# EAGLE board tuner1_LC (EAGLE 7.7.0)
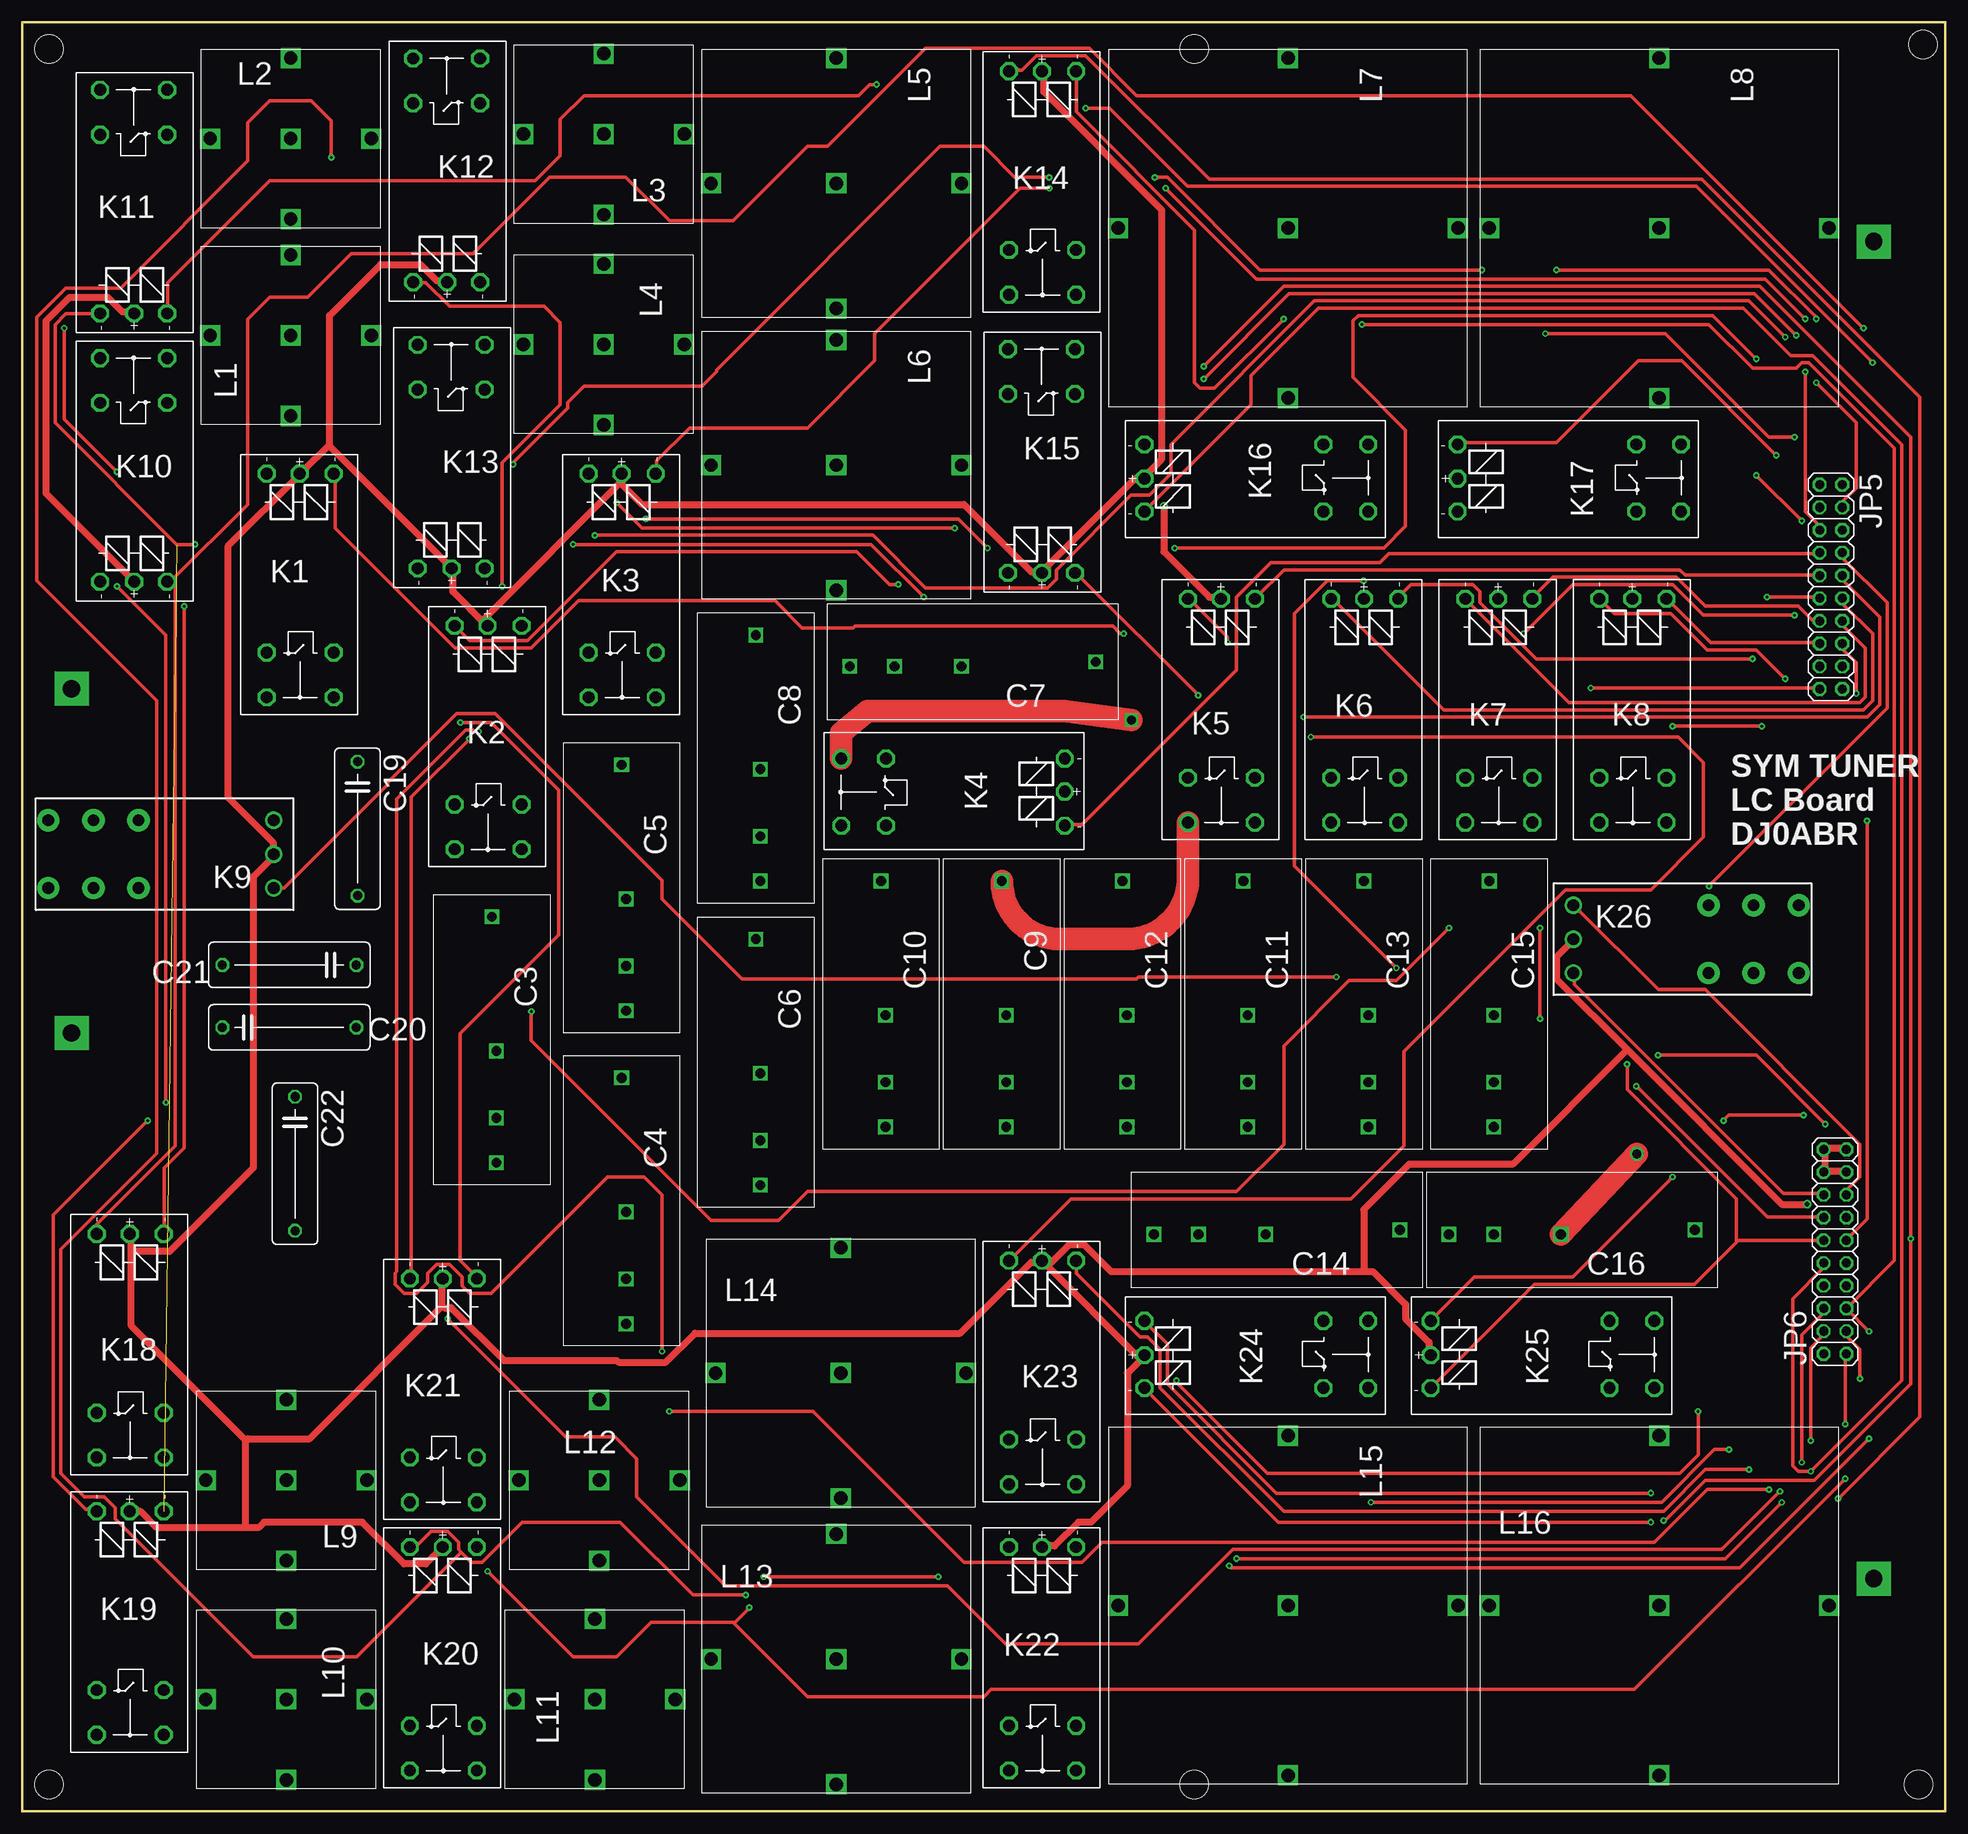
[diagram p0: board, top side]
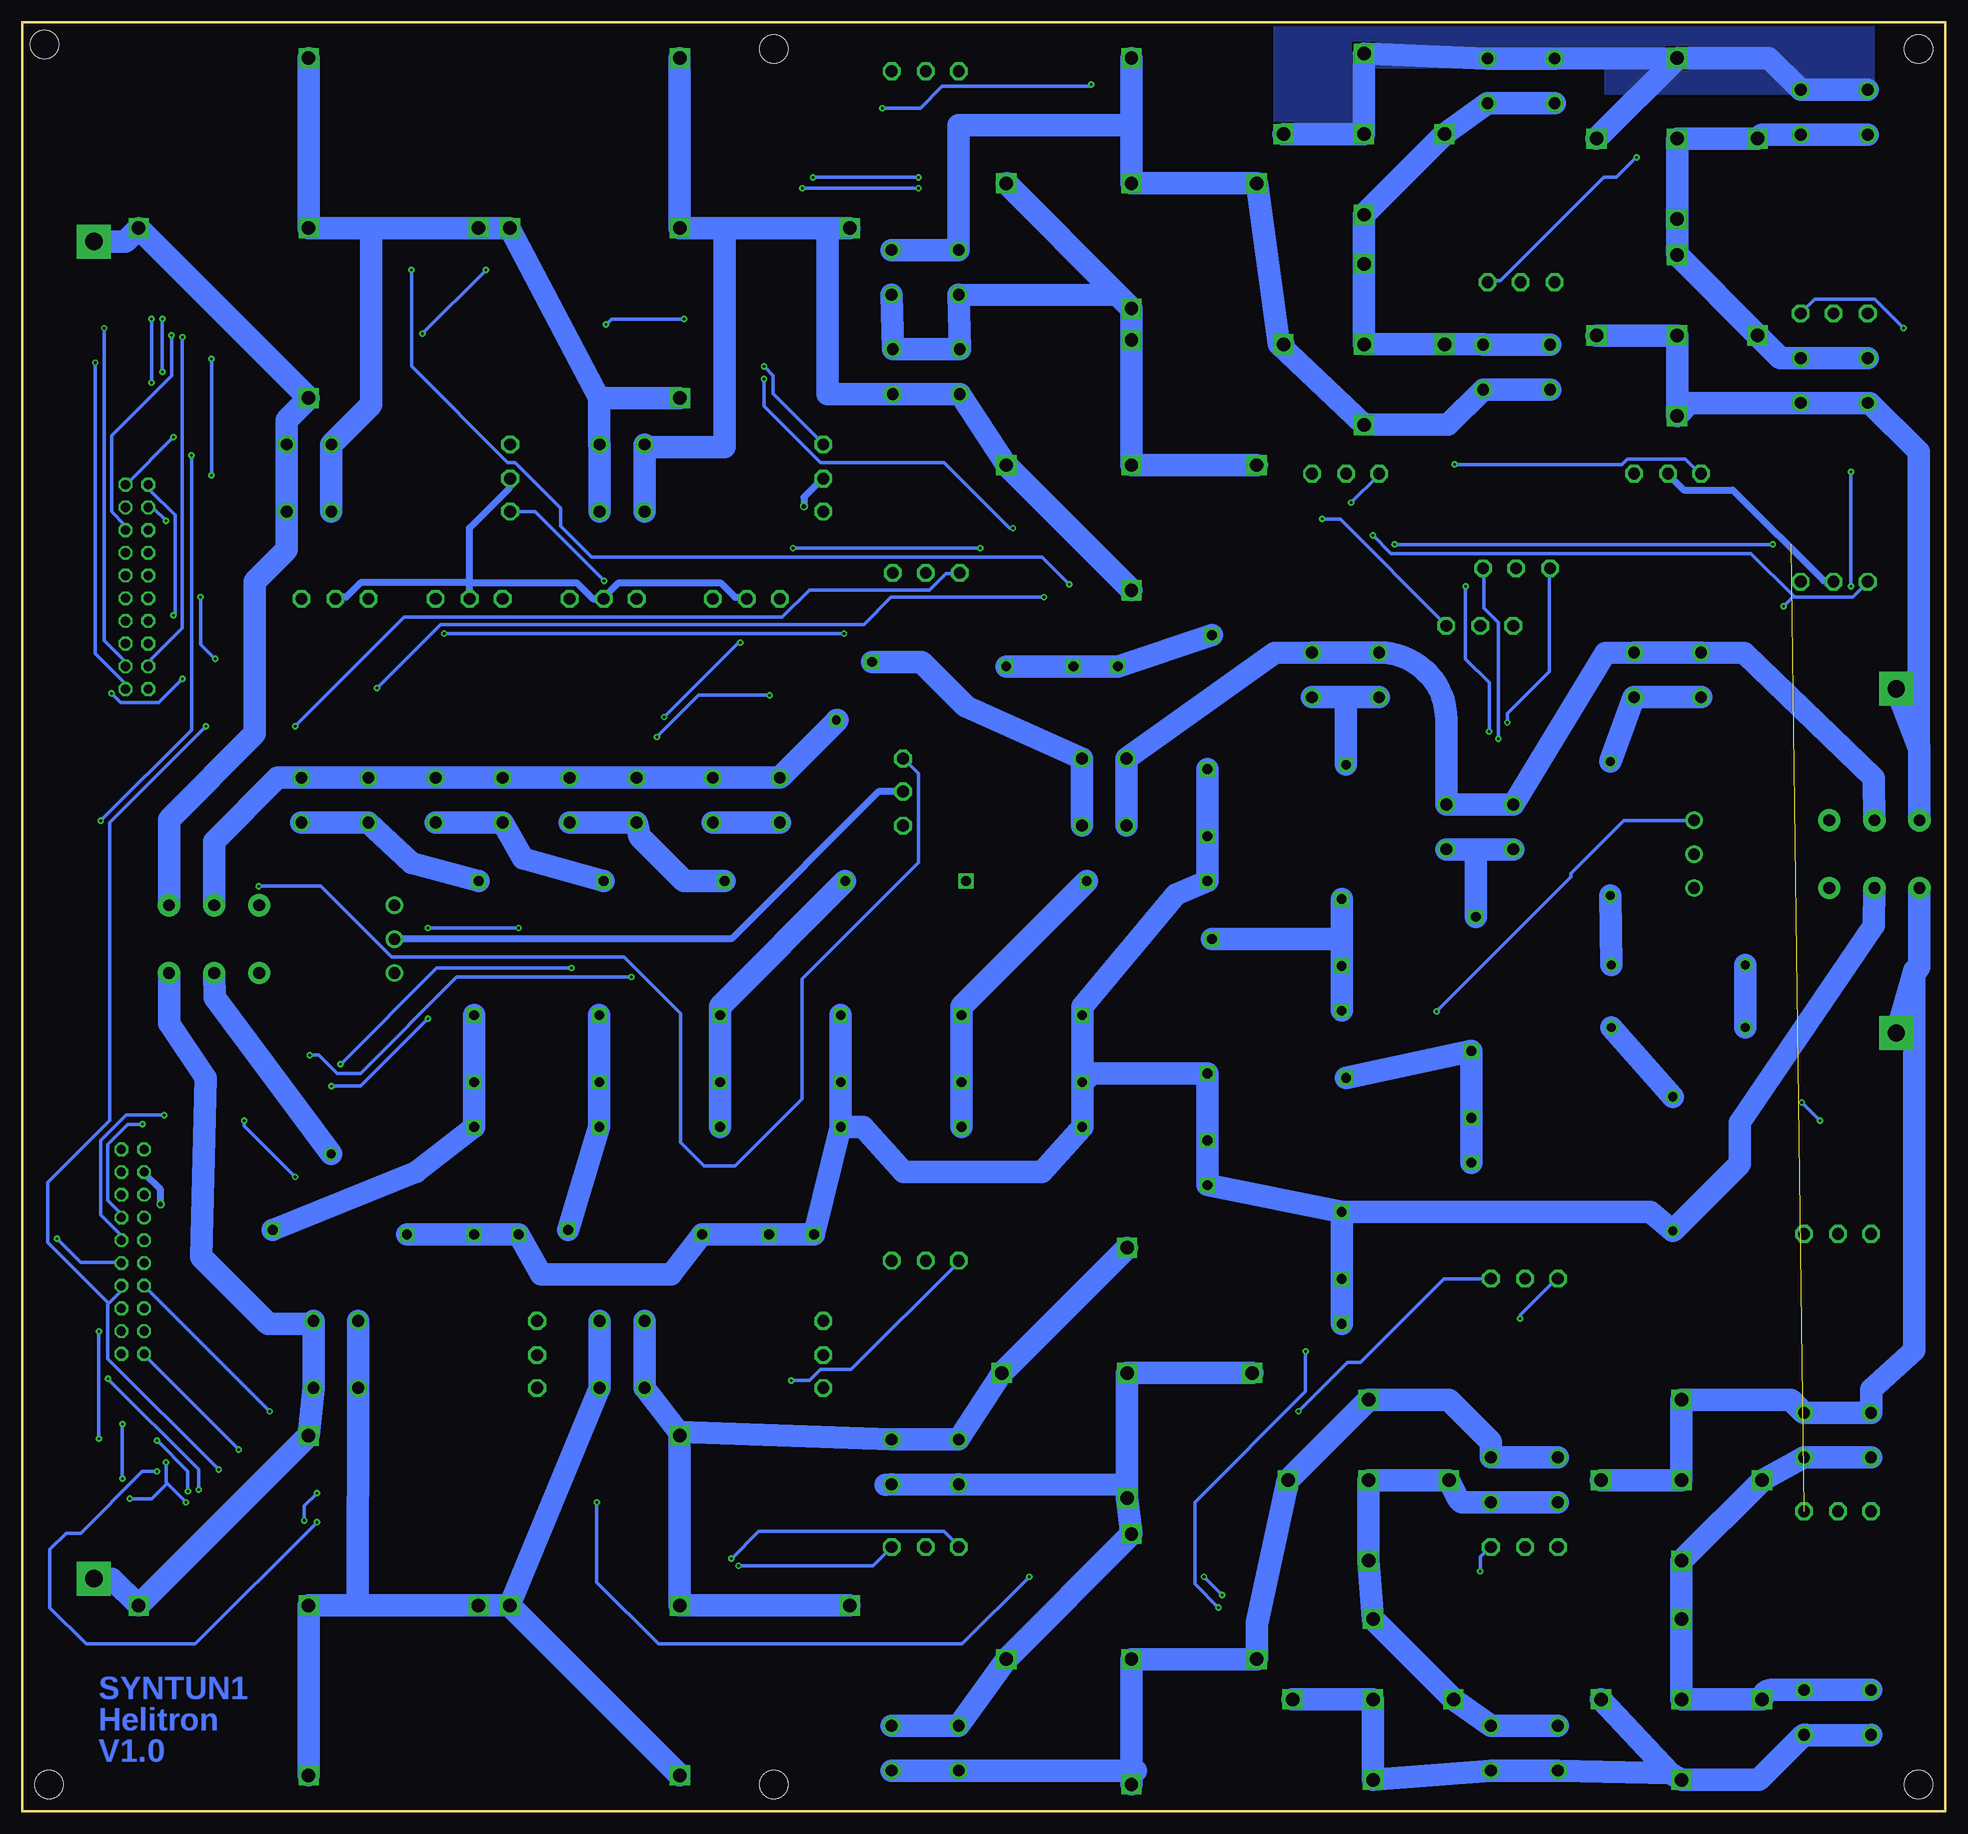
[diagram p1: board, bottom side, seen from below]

Size 215 x 200 mm. Coordinates in mm from the lower left corner, seen from the top.
Outline: 0,0 215,0 215,200 0,200 0,0
Copper layers (1*16): Top 0.035mm / dielectric 1.5mm / Bottom 0.035mm
Design rules "default *": minimum track width 16mil, minimum drill 0.3mm, track to track 16mil, track to pad 16mil, pad to pad 16mil, via to via 16mil, smd to smd 0mil, copper to edge 10mil, drill to drill 8mil, minimum pad ring 10mil, minimum via ring 8mil, stop-mask expansion 4mil, vias tented up to drill 0mil, thermal gap 10mil
Net classes: 1 Supply: width 0.762 mm, drill 0.5 mm; 2 HF: width 2.5 mm, drill 1 mm, clearance 2.5 mm
Holes 3.2 mm at 3,3 3,197 212.5,197.5 212,3 131,3 131,197

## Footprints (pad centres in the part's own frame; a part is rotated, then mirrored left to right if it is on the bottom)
C_FKP_MULTI = drill 1.1 square: 1 0,0; 2A 15,0.5; 2B 22.5,0.5; 2C 27.5,0.5
C150-054X183 = drill 1.016 octagon: 1 -7.493,0; 2 7.493,0
THICKPIN = drill 1.93 pad 3.81 square: 1 0,0
2X10 = drill 1.016 octagon: 1 -11.43,-1.27; 2 -11.43,1.27; 3 -8.89,-1.27; 4 -8.89,1.27; 5 -6.35,-1.27; 6 -6.35,1.27; 7 -3.81,-1.27; 8 -3.81,1.27; 9 -1.27,-1.27; 10 -1.27,1.27; 11 1.27,-1.27; 12 1.27,1.27; 13 3.81,-1.27; 14 3.81,1.27; 15 6.35,-1.27; 16 6.35,1.27; 17 8.89,-1.27; 18 8.89,1.27; 19 11.43,-1.27; 20 11.43,1.27
G2RLK1A = drill 1.321 octagon: 1 -2.54,-3.683; 2 -2.54,3.81; 3 -2.54,0; P 17.45,-3.683; P@ 17.45,3.81; S 22.454,-3.683; S@ 22.454,3.81
RT424 = drill 1.3 pad 2.5: 11 7.56,-3.78; 12 2.52,-3.78; 14 12.6,-3.78; 21 7.56,3.78; 22 2.52,3.78; 24 12.6,3.78 | drill 1.3: A1 -12.6,-3.78; A2 -12.6,3.78; A3 -12.6,0
L_D20 = drill 1.5 square: 1A 1,0; 1B 10,0; 1C 10,-9; 2A 19,0; 2B 10,9
L_D30 = drill 1.5 square: 1A 1,0; 1B 15,0; 1C 15,-14; 2A 29,0; 2B 15,14
L_D40 = drill 1.5 square: 1A 1,0; 1B 20,0; 1C 20,-19; 2A 39,0; 2B 20,19

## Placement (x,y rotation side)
C3  100p  [C_FKP_MULTI]  52.5,100 270 top
C4  100p  [C_FKP_MULTI]  67,82 270 top
C5  150p  [C_FKP_MULTI]  67,117 270 top
C6  220p  [C_FKP_MULTI]  82,97.5 270 top
C7  330p  [C_FKP_MULTI]  120,128.5 180 top
C8  330p  [C_FKP_MULTI]  82,131.5 270 top
C9  680p  [C_FKP_MULTI]  109.5,104 270 top
C10  680p  [C_FKP_MULTI]  96,104 270 top
C11  1n  [C_FKP_MULTI]  136.5,104 270 top
C12  1n5  [C_FKP_MULTI]  123,104 270 top
C13  1n5  [C_FKP_MULTI]  150,104 270 top
C14  4n7  [C_FKP_MULTI]  154,65 180 top
C15  3n3  [C_FKP_MULTI]  164,104 270 top
C16  4n7  [C_FKP_MULTI]  187,65 180 top
C19  100p  [C150-054X183]  37.47,109.86 270 top
C20  100p  [C150-054X183]  29.84,94.61 180 top
C21  100p  [C150-054X183]  29.84,87.63 0 top
C22  100p  [C150-054X183]  30.48,72.39 270 top
JP1  [THICKPIN]  5.5,125.5 0 top
JP2  [THICKPIN]  5.5,87 0 top
JP3  [THICKPIN]  207,175.5 0 top
JP4  [THICKPIN]  207,26 0 top
JP5  [2X10]  202.2,136.89 270 top
JP6  [2X10]  202.66,62.56 90 top
K1  G5RLK1AEDC12  [G2RLK1A]  31,147 270 top
K2  G5RLK1AEDC12  [G2RLK1A]  52,130 270 top
K3  G5RLK1AEDC12  [G2RLK1A]  67,147 270 top
K4  G5RLK1AEDC12  [G2RLK1A]  114,114 180 top
K5  G5RLK1AEDC12  [G2RLK1A]  134,133 270 top
K6  G5RLK1AEDC12  [G2RLK1A]  150,133 270 top
K7  G5RLK1AEDC12  [G2RLK1A]  165,133 270 top
K8  G5RLK1AEDC12  [G2RLK1A]  180,133 270 top
K9  RT424F12  [RT424]  15.5,107 180 top
K10  [G2RLK1A]  12.5,140 90 top
K11  [G2RLK1A]  12.5,170 90 top
K12  [G2RLK1A]  47.5,173.5 90 top
K13  [G2RLK1A]  48,141.5 90 top
K14  [G2RLK1A]  114,192 270 top
K15  [G2RLK1A]  114,141 90 top
K16  [G2RLK1A]  128,149 0 top
K17  [G2RLK1A]  163,149 0 top
K18  [G2RLK1A]  12,62 270 top
K19  [G2RLK1A]  12,31 270 top
K20  [G2RLK1A]  47,27 270 top
K21  [G2RLK1A]  47,57 270 top
K22  [G2RLK1A]  114,27 270 top
K23  [G2RLK1A]  114,59 270 top
K24  [G2RLK1A]  128,51 0 top
K25  [G2RLK1A]  160,51 0 top
K26  RT424F12  [RT424]  186,97.5 0 top
L1  187nH  [L_D20]  30,155 90 top
L2  375nH  [L_D20]  20,187 0 top
L3  750nH  [L_D20]  75,187.5 180 top
L4  1,5uH  [L_D20]  65,174 270 top
L5  3uH  [L_D30]  91,197 270 top
L6  6uH  [L_D30]  91,165.5 270 top
L7  12uH  [L_D40]  141.5,197 270 top
L8  24uH  [L_D40]  183,197 270 top
L9  187nH  [L_D20]  39.5,37 180 top
L10  375nH  [L_D20]  29.5,22.5 270 top
L11  750nH  [L_D20]  64,2.5 90 top
L12  1,5uH  [L_D20]  54.5,37 0 top
L13  3uH  [L_D30]  76,17 0 top
L14  6uH  [L_D30]  76.5,49 0 top
L15  12uH  [L_D40]  141.5,43 270 top
L16  24uH  [L_D40]  163,23 0 top

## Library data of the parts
C3-C16 L1-L16 = km_HF
C19-C22 = rcl
JP1-JP4 = km
JP5 JP6 = pinhead
K1-K8 K10-K25 = km; OC_FARNELL: unknown; OC_NEWARK: unknown
K9 K26 = relay; OC_FARNELL: unknown; OC_NEWARK: unknown

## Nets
+12V [Supply]: JP6.17 JP6.18 JP6.19 JP6.20 K1.3 K2.3 K3.3 K4.3 K5.3 K6.3 K7.3 K8.3 K9.A3 K10.3 K11.3 K12.3 K13.3 K14.3 K15.3 K16.3 K17.3 K18.3 K19.3 K20.3 K21.3 K22.3 K23.3 K24.3 K25.3 K26.A3
N$1 [HF]: C19.1 K1.S K1.S@
N$3 [HF]: C3.1 K2.S K2.S@
N$4 [HF]: C3.2A C3.2B C3.2C C4.1
N$5 [HF]: C5.1 K3.S K3.S@
N$6 [HF]: C5.2A C5.2B C5.2C C6.1
N$7 [HF]: C7.1 K4.P K4.P@
N$8 [HF]: C7.2A C7.2B C7.2C C8.1
N$9 [HF]: C9.1 K5.S K5.S@
N$10 [HF]: C9.2A C9.2B C9.2C C10.1
N$11 [HF]: C11.1 K6.S K6.S@
N$12 [HF]: C11.2A C11.2B C11.2C C12.1
N$13 [HF]: C13.1 K7.S K7.S@
N$14 [HF]: C13.2A C13.2B C13.2C C14.1
N$15 [HF]: C4.2A C4.2B C4.2C C6.2A C6.2B C6.2C C8.2A C8.2B C8.2C C10.2A C10.2B C10.2C C12.2A C12.2B C12.2C C14.2A C14.2B C14.2C C16.2A C16.2B C16.2C C22.2 K9.21 K26.11
N$16 [HF]: C15.1 K8.S K8.S@
N$17 [HF]: C15.2A C15.2B C15.2C C16.1
N$18 [HF]: K22.P K22.P@ K23.S K23.S@ L13.2A L13.2B L14.1A L14.1B L14.1C
N$19 [HF]: JP1.1 K9.14 K10.P K10.P@ L1.1A L1.1B L1.1C
N$20 [HF]: K11.S K11.S@ K12.S K12.S@ L2.2A L2.2B L3.1A L3.1B L3.1C
N$21 [HF]: K10.S K10.S@ K11.P K11.P@ L1.2A L1.2B L2.1A L2.1B L2.1C
N$22 [HF]: K1.P K1.P@ K2.P K2.P@ K3.P K3.P@ K4.S K4.S@ K5.P K5.P@ K6.P K6.P@ K7.P K7.P@ K8.P K8.P@ K9.11 K26.21
N$23 [HF]: K20.P K20.P@ K21.S K21.S@ L11.2A L11.2B L12.1A L12.1B L12.1C
N$24 [HF]: K12.P K12.P@ K13.S K13.S@ L3.2A L3.2B L4.1A L4.1B L4.1C
N$25 [HF]: K13.P K13.P@ K14.P K14.P@ L4.2A L4.2B L5.1A L5.1B L5.1C
N$26 [HF]: K14.S K14.S@ K15.S K15.S@ L5.2A L5.2B L6.1A L6.1B L6.1C
N$27 [HF]: K15.P K15.P@ K16.P K16.P@ L6.2A L6.2B L7.1A L7.1B L7.1C
N$28 [HF]: K16.S K16.S@ K17.P K17.P@ L7.2A L7.2B L8.1A L8.1B L8.1C
N$29 [HF]: JP3.1 K17.S K17.S@ K26.24 L8.2A L8.2B
N$30 [HF]: K23.P K23.P@ K24.P K24.P@ L14.2A L14.2B L15.1A L15.1B L15.1C
N$33: C19.2 C20.1
N$34: C20.2 C21.1
N$35: C21.2 C22.1
N$83 [HF]: JP4.1 K25.S K25.S@ K26.14 L16.2A L16.2B
N$84 [HF]: JP2.1 K9.24 K18.P K18.P@ L9.1A L9.1B L9.1C
N$85 [HF]: K18.S K18.S@ K19.P K19.P@ L9.2A L9.2B L10.1A L10.1B L10.1C
N$86 [HF]: K19.S K19.S@ K20.S K20.S@ L10.2A L10.2B L11.1A L11.1B L11.1C
N$88 [HF]: K21.P K21.P@ K22.S K22.S@ L12.2A L12.2B L13.1A L13.1B L13.1C
N$91 [HF]: K24.S K24.S@ K25.P K25.P@ L15.2A L15.2B L16.1A L16.1B L16.1C
REL1: JP5.1 K1.2
REL2: JP5.2 K1.1
REL3: JP5.3 K2.2
REL4: JP5.4 K2.1
REL5: JP5.5 K3.2
REL6: JP5.6 K3.1
REL7: JP5.7 K4.2
REL8: JP5.8 K4.1
REL9: JP5.9 K5.2
REL10: JP5.10 K5.1
REL11: JP5.11 K6.2
REL12: JP5.12 K6.1
REL13: JP5.13 K7.2
REL14: JP5.14 K7.1
REL15: JP5.15 K8.2
REL16: JP5.16 K8.1
REL17: JP5.17 K10.2 K18.2
REL18: JP5.18 K10.1 K18.1
REL19: JP5.19 K11.2 K19.2
REL20: JP5.20 K11.1 K19.1
REL21: JP6.1 K12.2 K20.2
REL22: JP6.2 K12.1 K20.1
REL23: JP6.3 K13.2 K21.2
REL24: JP6.4 K13.1 K21.1
REL25: JP6.5 K14.2 K22.2
REL26: JP6.6 K14.1 K22.1
REL27: JP6.7 K15.2 K23.2
REL28: JP6.8 K15.1 K23.1
REL29: JP6.9 K16.2 K24.2
REL30: JP6.10 K16.1 K24.1
REL31: JP6.11 K17.2 K25.2
REL32: JP6.12 K17.1 K25.1
REL33: JP6.13 K9.A2
REL34: JP6.14 K9.A1
REL35: JP6.15 K26.A2
REL36: JP6.16 K26.A1

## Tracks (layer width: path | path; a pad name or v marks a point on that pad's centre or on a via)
+12V  (via drill 0.5)
  Top 0.762: K22.3 114.2,29.67 115.42,29.67 118.06,32.31 119.48,32.31 123.55,36.37 123.55,48.97 125.37,50.8 K24.3 124.97,50.6 114.2,61.37 K23.3 | 149.96,60.35 121.72,60.35 118.67,63.4 117.04,63.4 114.81,61.16 K23.3 | 149.96,60.35 150.98,60.35 154.63,56.69 154.63,55.07 157.28,52.43 157.28,51 K25.3 | JP6.17 203.81,71.53 201.57,71.53 JP6.18 201.57,71.93 201.57,73.97 JP6.20 201.78,74.17 203.81,74.17 JP6.19 | v199.54,67.87 196.7,67.87 179.43,85.14 | 179.43,85.14 171.5,93.07 171.5,95.5 173.33,97.33 K26.A3 | 149.96,60.35 149.96,67.26 155.04,72.34 166.62,72.34 179.43,85.14 | K14.3 114.2,194.46 114.2,192.23 127.41,179.02 127.41,151.18 125.58,149.35 K16.3 125.37,148.95 124.36,148.95 114.61,139.19 114.61,138.99 114.2,138.58 K15.3 113.79,138.58 112.78,138.58 105.26,146.1 69.29,146.1 66.85,148.54 | v127.61,145.9 127.61,140.82 132.69,135.74 133.91,135.74 K5.3 | 24.99,31.7 26.42,31.7 27.03,32.31 38,32.31 42.67,27.64 45.11,27.64 46.94,29.46 K20.3 | 24.99,31.7 15.04,31.7 13.21,33.53 12.19,33.53 K19.3 | 12.19,62.59 12.19,54.25 24.99,41.45 | 12.19,62.59 12.19,64.41 K18.3 | 24.99,31.7 24.99,41.45 | 46.94,56.49 46.94,59.54 K21.3 | 46.94,56.49 32.11,41.66 25.2,41.66 24.99,41.45 | 66.85,148.54 66.85,149.35 K3.3 | 66.85,148.54 51.61,133.3 K2.3 51.82,132.69 48.16,136.35 48.16,138.79 K13.3 47.75,139.19 34.34,152.6 34.34,152.81 | K11.3 12.39,167.64 11.18,167.64 9.55,169.27 5.28,169.27 2.64,166.62 2.64,147.32 12.39,137.57 K10.3 | 34.34,152.81 34.34,167.23 40.03,172.92 44.5,172.92 46.33,171.09 47.35,171.09 K12.3 | 34.34,152.81 31.29,149.76 K1.3 30.89,149.35 22.96,141.43 22.96,113.39 28.04,108.31 28.04,107.09 K9.A3 28.04,106.68 25.81,104.44 25.81,71.93 16.46,62.59 12.19,62.59
  Top 0.762: K23.3 113.79,61.37 112.78,61.37 104.85,53.44 75.18,53.44 71.93,50.19 66.65,50.19 66.45,50.39 53.85,50.39 47.95,56.29 47.14,56.29 46.94,56.49
  Bottom 0.762: K26.A3 173.33,97.54 135.74,97.54 119.28,114 116.64,114 K4.3 | v199.54,67.87 199.54,69.49 201.37,71.32 JP6.18 | K5.3 134.11,135.74 135.33,135.74 136.96,137.36 148.34,137.36 149.96,135.74 K6.3 150.37,135.53 151.18,135.53 153.01,137.36 165,137.36 | 165,137.36 165,135.74 K7.3 | 165,137.36 165,143.46 160.53,147.93 160.53,148.95 K17.3 | 165,137.36 177.19,137.36 178.82,135.74 179.83,135.74 K8.3 | v127.61,145.9 127.61,146.91 125.58,148.95 K16.3 | K10.3 12.6,137.57 13.61,137.57 23.77,147.73 29.26,147.73 30.89,149.35 K1.3
N$1
  Bottom 2.5: K1.S K1.S@ C19.1
N$3
  Bottom 2.5: K2.S 52.5,107.52 | 52.5,107.52 55,107.5 K2.S@ | C3.1 52.5,107.52
N$4
  Bottom 2.5: C3.2C C3.2B C3.2A C4.1
N$5
  Bottom 2.5: K3.S@ 67,124.55 | 67,124.55 K3.S | C5.1 67,124.55
N$6
  Bottom 2.5: C5.2A 67.5,97.5 | 67.5,97.5 C5.2B C5.2C | C6.1 67.5,97.5
N$7
  Bottom 2.5: K4.P@ K4.P 109.5,123.5 114.5,128.5 C7.1
N$8
  Bottom 2.5: C8.1 C7.2C C7.2B C7.2A
N$9
  Top 2.5: K5.S 130.32,104.32 arc-90 123.5,97.5 116,97.5 arc-90 C9.1
  Bottom 2.5: K5.S K5.S@
N$10
  Bottom 2.5: C10.1 110,90 C9.2A C9.2B C9.2C
N$11
  Bottom 2.5: C11.1 141,104 146,109 K6.S K6.S@
N$12
  Bottom 2.5: C12.1 137,90 C11.2A C11.2B C11.2C
N$13
  Bottom 2.5: C13.1 159,106.5 K7.S K7.S@
N$14
  Bottom 2.5: C13.2A C13.2B C13.2C C14.1
N$15  (via drill 1)
  Top 2.5: C16.2A v180.5,73.5
  Bottom 2.5: C8.2A C8.2B C8.2C 86,102.5 96.5,90 C10.2A C10.2B | C10.2B 95.5,82.5 C6.2A C6.2B C6.2C C4.2A | C10.2B C10.2C 101,71.5 116.5,71.5 121,76.5 C12.2C | C12.2C C12.2B C12.2A | C16.2A C16.2B C16.2C 157,60 142.5,60 C14.2A C14.2B C14.2C C12.2C | C4.2A C4.2B C4.2C | C4.2A 33,67 C22.2 23,72.38 23,77 8,99 K9.21 | v180.5,73.5 193.5,91 K26.11
N$16
  Bottom 2.5: C15.1 171.5,106 K8.S K8.S@
N$17
  Bottom 2.5: C15.2A C15.2B C15.2C 171,71.5 C16.1
N$18
  Bottom 2.5: L14.1A L14.1B 91.5,36.5 | 91.5,36.5 L14.1C L13.2B L13.2A K22.P K22.P@ | 91.5,36.5 K23.S 118.5,36.5 K23.S@
N$19
  Bottom 2.5: JP1.1 3,119 | 3,119 3,152 8.45,157.45 K10.P@ K10.P 28.55,157.45 L1.1A L1.1B L1.1C | K9.14 2.9,118.9 arc-90 3,119
N$20
  Bottom 2.5: K11.S@ K11.S 19.73,196 L2.2B | L2.2B L2.2A | L2.2B K12.S@ K12.S 64.5,196.5 L3.1C L3.1B L3.1A
  pour Bottom: 8,199.5 8,192.5 16,192.5 16,192 38,192 38,195 64.5,195 64.5,186.5 75,186.5 75,199.5
N$21
  Bottom 2.5: K11.P@ K11.P 20.55,187.45 L2.1A L2.1B L2.1C L1.2A L1.2B 18.45,162.45 K10.S K10.S@
N$22  (via drill 1)
  Top 2.5: v124,122 116.5,123 94.5,123 91.55,120.55 K4.S
  Bottom 2.5: K4.S@ K4.S 75,129.5 K3.P@ K3.P arc90 55.81,122.04 K2.P@ K2.P 38,129.5 K1.P@ K1.P 22.5,129.5 8,115.5 K9.11 | v124,122 123.87,122 K5.P K5.P@ K6.P K6.P@ K7.P K7.P@ K8.P K8.P@ 186.45,115.55 193.56,108.44 K26.21
N$23
  Bottom 2.5: K20.P K20.P@ L11.2B L11.2A L12.1C L12.1B L12.1A 54.5,35 54.05,34.55 K21.S@ K21.S
N$24
  Bottom 2.5: K12.P@ K12.P L3.2A L3.2B L4.1A L4.1B L4.1C 51.73,164 K13.S K13.S@
N$25
  Bottom 2.5: 74.5,164 L4.2A 55.63,155 K13.P K13.P@ | 74.5,164 L4.2B | 74.5,164 L5.1C L5.1B 91,188.5 | L5.1A 91,188.5 | K14.P@ K14.P 110.32,188.5 91,188.5
N$26
  Bottom 2.5: L5.2B 92.5,169.5 | 92.5,169.5 L5.2A L6.1A L6.1B L6.1C | K14.S@ K15.S K15.S@ K14.S 92.5,169.5
N$27
  Bottom 2.5: L6.2A L6.2B K15.P@ K15.P 125,158.45 125,177 L7.1C 136.5,177 | L7.1A L7.1B 136.5,177 | 136.5,177 136.5,152.5 145.45,152.5 | K16.P@ 145.45,152.5 | 145.45,152.5 K16.P
N$28
  Bottom 2.5: K16.S K16.S@ 150.5,152.81 150.5,158 | 150.5,158 L7.2A | 150.5,158 L7.2B L8.1C 176,177 | 176,177 L8.1B L8.1A | 176,177 176,157.26 K17.P@ K17.P
N$29
  Bottom 2.5: JP3.1 203.5,175.5 L8.2B L8.2A 185.45,155.55 K17.S@ K17.S 185.45,141.05 189,137.5 189,120.5 198.6,110.9 K26.24
N$30
  Bottom 2.5: L14.2B L14.2A K23.P K23.P@ 141.62,42.41 | 141.62,42.41 K24.P K24.P@ | L15.1C L15.1B L15.1A 141.62,42.41
N$33
  Bottom 2.5: C19.2 C20.1
N$34
  Bottom 2.5: C20.2 C21.1
N$35
  Bottom 2.5: C22.1 C21.2
N$83
  Bottom 2.5: JP4.1 205,26 L16.2A L16.2B K25.S K25.S@ 182.76,54.5 187.5,54.5 195,62 194.5,82 198.6,88.1 K26.14
N$84
  Bottom 2.5: JP2.1 3.5,94 | 3.5,94 3.5,51.5 8.32,47.18 K18.P K18.P@ 17.26,46 L9.1C L9.1B L9.1A | K9.24 2.9,94.6 arc90 3.5,94
N$85
  Bottom 2.5: K18.S K18.S@ L9.2A L9.2B L10.1A L10.1B L10.1C arc90 19.45,13.55 K19.P@ K19.P
N$86
  Bottom 2.5: 30.75,4.25 L10.2A 20.86,3.5 K19.S@ 15.55,8.55 15.5,8.5 8.36,8.5 K19.S | 30.75,4.25 L10.2B | L11.1C L11.1B L11.1A K20.S@ K20.S 30.75,4.25
N$88
  Bottom 2.5: K21.P K21.P@ 50.81,41.31 55.5,46 L12.2B L12.2A 77,21 L13.1A L13.1B 91,4.5 | 91,4.5 L13.1C | K22.S@ K22.S 90.5,4.5 91,4.5
N$91
  Bottom 2.5: 177.5,23 L16.1A L15.2B | 177.5,23 L16.1B L16.1C | L15.2A L15.2B | L15.2B K24.S K24.S@ | K25.P@ K25.P 177.5,23
REL1  (via drill 0.3)
  Top 0.406: v198.12,133.71 187.96,133.71 184.51,137.16 173.33,137.16 v167.84,131.67 | v123.14,131.67 122.73,131.67 121.92,132.49 93.07,132.49 92.86,132.28 87.17,132.28 84.12,135.33 62.18,135.33 56.9,130.05 48.36,130.05 34.95,143.46 34.95,149.35 K1.2
  Bottom 0.406: v198.12,133.71 197.92,133.91 197.92,144.88 200.76,147.73 200.76,148.13 JP5.1 | v123.14,131.67 v167.84,131.67
REL2  (via drill 0.3)
  Top 0.406: v198.12,153.62 195.28,153.62 183.69,165.2 v170.28,165.2 | v163.17,172.31 138.38,172.31 128.02,182.68 v126.59,182.68 | v114.81,182.68 110.95,182.68 107.49,186.13 102.62,186.13 77.62,161.14 77.62,160.93 76,159.31 62.79,159.31 60.96,157.48 60.96,156.87 54.86,150.77 v54.86,150.57
  Bottom 0.406: v198.12,153.62 203.4,148.34 JP5.2 | v163.17,172.31 v170.28,165.2 | v114.81,182.68 v126.59,182.68 | v54.86,150.57 36.17,150.57 35.56,151.18 29.06,151.18 27.43,149.56 K1.1
REL3  (via drill 0.3)
  Top 0.406: v193.85,149.35 v198.93,144.27 | v193.85,162.36 188.98,167.23 149.35,167.23 148.74,166.62 148.74,160.32 154.63,154.43 154.63,143.66 152.2,141.22 v128.83,141.22 | v107.9,141.22 104.65,144.47 v69.7,144.47
  Bottom 0.406: v198.93,144.27 200.35,145.69 200.76,145.69 JP5.3 | v193.85,162.36 v193.85,149.35 | v107.9,141.22 v128.83,141.22 | v69.7,144.47 67.67,144.47 55.88,132.69 K2.2
REL4  (via drill 0.3)
  Top 0.406: v200.56,159.72 205.03,155.25 205.03,147.93 203.61,146.51 203.61,145.9 JP5.4 | v200.56,166.83 200.56,167.03 195.28,172.31 v171.5,172.31 | v97.94,137.16 96.93,137.16 93.27,140.82 66.45,140.82 56.49,130.86 49.99,130.86 48.36,132.49 K2.1
  Bottom 0.406: v200.56,166.83 v200.56,159.72 | v171.5,172.31 171.5,161.54 160.73,150.77 159.92,150.77 154.84,145.69 154.84,143.66 151.38,140.21 100.99,140.21 v97.94,137.16
REL5  (via drill 0.3)
  Top 0.406: v199.34,160.93 199.34,145.29 200.76,143.87 200.76,143.26 JP5.5 | v199.34,166.83 194.87,171.3 137.97,171.3 v127.81,181.46 | v114.81,181.46 111.56,181.46 95.3,165.2 95.3,162.15 87.78,154.63 74.57,154.63 70.92,150.98 70.92,149.56 K3.2
  Bottom 0.406: v199.34,166.83 v199.34,160.93 | v114.81,181.46 v127.81,181.46
REL6  (via drill 0.3)
  Top 0.406: v198.32,165 193.65,169.67 141.63,169.67 v132.08,160.12 | v104.24,143.46 69.29,143.46 v66.45,146.3
  Bottom 0.406: v198.32,165 198.32,160.53 205.03,153.82 205.03,145.29 203.61,143.87 203.61,143.26 JP5.6 | v132.08,160.12 132.08,157.07 125.78,150.77 111.96,150.77 104.65,143.46 v104.24,143.46 | v66.45,146.3 63.4,149.35 K3.1
REL7
  Top 0.406: JP5.7 200.76,140.61 152.81,140.61 151.79,139.6 139.6,139.6 135.74,135.74 135.74,127.61 118.47,110.34 116.64,110.34 K4.2
REL8  (via drill 0.3)
  Top 0.406: v188.57,103.43 208.48,123.34 208.48,135.13 203.61,140 203.61,140.61 JP5.8
  Bottom 0.406: v188.57,103.43 181.66,103.43 173.74,95.5 147.73,95.5 141.43,89.2 141.43,74.78 138.79,72.14 135.33,72.14 127.81,79.65 127.81,93.07 114.81,106.07 114.81,116.03 116.43,117.65 K4.1
REL9
  Top 0.406: JP5.9 200.76,138.18 185.93,138.18 185.32,138.79 141.02,138.79 137.97,135.74 K5.2
REL10  (via drill 0.3)
  Top 0.406: v143.26,122.33 206.25,122.33 207.67,123.75 207.67,133.5 203.61,137.57 203.61,137.97 JP5.10 | v134.72,130.66 134.72,131.27 130.45,135.53 K5.1
  Bottom 0.406: v143.26,122.33 134.93,130.66 v134.72,130.66
REL11  (via drill 0.3)
  Top 0.406: v195.07,135.74 200.76,135.74 JP5.11 | v193.45,128.83 169.27,128.83 162.97,135.13 162.97,136.35 162.15,137.16 155.25,137.16 153.82,135.74 K6.2
  Bottom 0.406: v195.07,135.74 195.07,130.45 v193.45,128.83
REL12
  Top 0.406: JP5.12 203.61,135.53 203.61,134.93 206.86,131.67 206.86,124.16 205.84,123.14 158.9,123.14 146.51,135.53 K6.1
REL13
  Top 0.406: JP5.13 200.76,133.1 200.15,133.1 198.53,134.72 188.16,134.72 184.91,137.97 171.09,137.97 168.86,135.74 K7.2
REL14
  Top 0.406: JP5.14 203.61,132.89 203.61,132.49 206.04,130.05 206.04,124.56 205.44,123.95 172.92,123.95 161.34,135.53 K7.1
REL15
  Top 0.406: JP5.15 200.76,130.66 188.77,130.66 183.9,135.53 K8.2
REL16  (via drill 0.3)
  Top 0.406: v205.03,124.97 205.03,128.42 203.61,129.84 203.61,130.45 JP5.16 | v197.1,126.59 193.85,129.84 188.37,129.84 184.3,133.91 178,133.91 176.38,135.53 K8.1
  Bottom 0.406: v205.03,124.97 204.01,123.95 199.75,123.95 v197.1,126.59
REL17  (via drill 0.3)
  Top 0.406: v197.1,164.79 193.04,168.86 144.47,168.86 128.42,152.81 128.42,149.56 125.98,147.12 123.95,147.12 115.62,138.79 115.62,137.77 114.61,136.75 100.99,136.75 95.1,142.65 v64.01,142.65 | v18.09,134.72 18.09,74.17 15.85,71.93 15.85,64.62 K18.2
  Bottom 0.406: v197.1,164.79 197.1,132.28 200.76,128.63 200.76,128.02 JP5.17 | v64.01,142.65 61.98,140.61 21.74,140.61 16.97,135.84 | 16.97,135.84 16.87,135.74 10.36,135.74 8.74,137.36 K10.2 | 16.97,135.84 v18.09,134.72
REL18  (via drill 0.3)
  Top 0.406: v205.84,165.81 179.83,191.82 124.56,191.82 119.28,197.1 100.99,197.1 90.02,186.13 87.78,186.13 79.45,177.8 72.34,177.8 67.46,182.68 58.93,182.68 50.39,174.14 36.78,174.14 31.9,169.27 27.64,169.27 25.2,166.83 25.2,146.1 16.66,137.57 16.26,137.57 K10.1 17.07,137.77 17.07,74.37 8.33,65.63 8.33,64.62 K18.1
  Bottom 0.406: v205.84,165.81 205.84,130.86 203.61,128.63 203.61,128.02 JP5.18
REL19  (via drill 0.3)  (1 unrouted)
  Top 0.406: v175.36,125.58 200.76,125.58 JP5.19 | v100.79,135.74 94.89,141.63 v61.57,141.63 | v19.3,141.63 17.27,141.63 3.66,155.25 3.66,166.22 4.88,167.44 8.53,167.44 K11.2
  Bottom 0.406: v175.36,125.58 168.25,132.69 120.9,132.69 117.86,135.74 v100.79,135.74 | v19.3,141.63 v61.57,141.63
REL20  (via drill 0.3)
  Top 0.406: v206.86,161.95 187.15,181.66 130.25,181.66 121.51,190.4 v118.87,190.4 | v95.5,193.04 94.69,193.04 93.47,191.82 62.79,191.82 60.15,189.18 60.15,185.12 57.3,182.27 27.64,182.27 16.26,170.89 16.26,167.64 K11.1 | v14.02,77.22 3.45,66.65 3.45,37.39 7.11,33.73 8.13,33.73 K19.1 | v16.05,79.25 16.05,131.47 v10.57,136.96 | v10.57,149.76 4.67,155.65 v4.67,165.81
  Bottom 0.406: v206.86,161.95 206.86,129.44 203.61,126.19 203.61,125.58 JP5.20 | v118.87,190.4 114.61,190.4 112.17,192.84 95.71,192.84 v95.5,193.04 | v16.05,79.25 v14.02,77.22 | v10.57,149.76 v10.57,136.96 | v4.67,165.81 7.92,169.06 14.63,169.06 16.05,167.64 K11.1
REL21  (via drill 0.3)
  Top 0.406: v203.81,43.28 203.81,51 JP6.1 | v203.81,37.19 180.24,13.61 108.31,13.61 107.49,12.8 87.78,12.8 79.55,21.03 | 79.55,21.03 79.45,21.13 70.31,21.13 66.45,17.27 61.57,17.27 v52.02,26.82 | v53.65,136.96 53.65,150.77 60.15,157.28 60.15,166.42 58.32,168.25 47.75,168.25 45.11,170.89 43.89,170.89 K12.2 | v51,120.7 50.6,120.7 50.39,120.9 49.58,120.9 41.86,113.18 41.86,60.35 41.66,60.15 41.66,58.93 42.67,57.91 44.09,57.91 45.31,59.13 45.31,60.15 46.33,61.16 47.75,61.16 49.17,59.74 49.17,58.73 49.99,57.91 52.43,57.91 65.43,70.92 69.49,70.92 71.53,68.89 v71.53,51.41 | 79.55,21.03 v81.28,22.76
  Bottom 0.406: v203.81,37.19 v203.81,43.28 | v52.02,26.82 52.02,28.45 51,29.46 K20.2 | v53.65,136.96 53.65,128.83 51,126.19 v51,120.7 | v71.53,51.41 71.53,46.94 83.92,34.54 83.92,25.4 v81.28,22.76
REL22  (via drill 0.3)
  Top 0.406: v190.81,40.44 189.18,40.44 183.29,34.54 v150.77,34.54 | v82.91,26.21 v102.41,26.21 | v80.87,24.18 74.98,24.18 66.85,32.31 55.88,32.31 51.41,27.84 50.19,27.84 49.07,28.96 | 49.07,28.96 48.77,29.26 48.77,30.07 47.55,31.29 45.72,31.29 44.09,29.67 43.48,29.67 K20.1 | v34.54,184.91 34.54,188.98 32.31,191.21 27.64,191.21 25.2,188.77 25.2,184.51 10.97,170.28 4.88,170.28 1.63,167.03 1.63,137.57 15.04,124.16 15.04,73.56 4.27,62.79 4.27,37.8 6.91,35.15 9.14,35.15 10.36,33.93 10.36,32.72 25.81,17.27 37.39,17.27 49.07,28.96
  Bottom 0.406: v190.81,40.44 201.37,51 JP6.2 | v150.77,34.54 150.77,25.6 143.87,18.69 109.93,18.69 v102.41,26.21 | v80.87,24.18 v82.91,26.21 | v34.54,184.91 36.78,182.68 38.2,182.68 49.78,171.09 51,171.09 K12.1
REL23  (via drill 0.3)
  Top 0.406: v205.44,48.36 205.44,51.61 204.01,53.03 204.01,53.65 JP6.3 | v195.28,35.97 188.37,35.97 182.47,30.07 120.7,30.07 118.47,27.84 105.26,27.84 88.39,44.7 v72.34,44.7 | v48.97,121.72 52.43,121.72 59.94,114.2 59.94,97.94 48.97,86.97 48.97,61.57 50.8,59.74 K21.2
  Bottom 0.406: v205.44,48.36 195.28,38.2 v195.28,35.97 | v72.34,44.7 66.85,50.19 65.43,50.19 56.08,59.54 51,59.54 K21.2 | v48.97,121.72 48.97,122.73 44.3,127.41 44.3,138.79 K13.2
REL24  (via drill 0.3)
  Top 0.406: v199.95,41.45 199.95,51.82 201.37,53.24 201.37,53.65 JP6.4 | v196.49,35.76 189.99,29.26 135.33,29.26 124.77,18.69 109.93,18.69 103.43,25.2 78.64,25.2 68.68,35.15 68.68,39.42 66.24,41.86 60.76,41.86 v47.55,55.07 | v49.99,119.89 43.48,113.39 43.48,59.74 K21.1
  Bottom 0.406: v199.95,41.45 196.49,38 v196.49,35.76 | v47.55,55.07 47.55,55.47 43.48,59.54 K21.1 | v49.99,119.89 49.99,132.89 51.61,134.52 51.61,138.79 K13.1
REL25  (via drill 0.3)
  Top 0.406: v206.45,53.65 204.01,56.08 JP6.5 204.01,56.29 209.3,61.57 209.3,152.4 199.75,161.95 198.93,161.95 198.32,161.34 193.45,161.34 188.57,166.22 v149.76,166.22 | v206.45,41.66 192.02,27.23 135.13,27.23 v134.93,27.43 | v141.02,166.83 133.3,159.11 131.67,159.11 131.06,159.72 131.06,176.78 117.86,189.99 117.86,194.46 K14.2
  Bottom 0.406: v206.45,41.66 v206.45,53.65 | v134.93,27.43 119.89,27.43 117.86,29.46 K22.2 | v141.02,166.83 149.15,166.83 v149.76,166.22
REL26  (via drill 0.3)
  Top 0.406: v198.93,39.01 198.93,53.24 201.37,55.68 201.37,56.08 JP6.6 | v196.7,34.54 190.4,28.25 v135.74,28.25 | v203,34.95 212.14,44.09 212.14,158.09 187.76,182.47 132.69,182.47 118.87,196.29 113.39,196.29 111.76,194.67 110.34,194.67 K14.1
  Bottom 0.406: v198.93,39.01 198.93,36.78 198.83,36.68 | v196.7,34.54 198.83,36.68 | v135.74,28.25 132.69,31.29 111.96,31.29 110.34,29.67 K22.1 | v203,34.95 200.56,34.95 198.83,36.68
REL27  (via drill 0.3)
  Top 0.406: v193.04,38.2 188.16,38.2 183.49,33.53 141.02,33.53 127.2,47.35 127.2,51.61 125.78,53.03 124.97,53.03 117.86,60.15 117.86,61.37 K23.2 | v194.46,121.31 v184.51,121.31
  Bottom 0.406: 205.33,56.79 205.44,56.69 205.44,50.6 v193.04,38.2 | 205.33,56.79 204.01,58.12 204.01,58.73 JP6.7 | v184.51,121.31 172.31,133.5 130.05,133.5 127,136.55 113.59,136.55 111.76,138.38 110.34,138.38 K15.2 | v194.46,121.31 205.23,110.54 205.23,77.22 212.14,70.31 212.14,63.6 205.33,56.79
REL28  (via drill 0.3)
  Top 0.406: v187.35,44.7 187.35,39.83 185.32,37.8 139.19,37.8 129.03,47.95 v129.03,48.16 | v131.47,124.77 117.86,138.38 K15.1 | v144.07,120.09 185.12,120.09 187.96,117.25 187.96,108.92 182.07,103.02 172.52,103.02 154.43,84.94 154.43,74.37 148.54,68.48 117.25,68.48 110.34,61.57 K23.1
  Bottom 0.406: v187.35,44.7 201.37,58.73 JP6.8 | v129.03,48.16 127,48.16 125.78,49.38 122.33,49.38 110.34,61.37 K23.1 | v131.47,124.77 139.4,124.77 v144.07,120.09
REL29  (via drill 0.3)
  Top 0.406: v183.49,32.51 183.69,32.51 188.16,36.98 200.35,36.98 211.12,47.75 v211.12,64.01 211.12,153.62 194.26,170.49 141.02,170.49 v132.08,161.54 | v182.07,35.56 140.21,35.56 128.02,47.75 128.02,52.22 125.58,54.66 K24.2
  Bottom 0.406: v211.12,64.01 208.48,61.37 204.01,61.37 JP6.9 | v183.49,32.51 183.49,34.14 v182.07,35.56 | v132.08,161.54 131.06,160.53 131.06,158.5 125.58,153.01 K16.2
REL30  (via drill 0.3)
  Top 0.406: v182.07,32.31 140.41,32.31 125.58,47.14 K24.1 | JP6.10 201.37,61.16 201.37,60.76 197.92,57.3 197.92,38.61 198.53,38 v199.95,38 210.11,48.16 210.11,152.81 200.15,162.76 197.71,162.76 192.43,168.05 144.88,168.05 137.36,160.53 137.36,157.28 125.58,145.49 K16.1
  Bottom 0.406: v199.95,38 201.57,38 208.48,31.09 210.11,31.09 211.94,29.26 211.94,22.76 207.87,18.69 195.68,18.69 v182.07,32.31
REL31  (via drill 0.3)
  Top 0.406: v199.14,77.83 190.81,77.83 v190.19,77.22 | v184.51,70.92 173.33,59.74 162.36,59.74 157.48,54.86 K25.2 | v196.09,151.59 185.52,162.15 180.65,162.15 171.5,153.01 160.53,153.01 K17.2 | v206.25,110.74 206.25,66.24 204.01,64.01 JP6.11
  Bottom 0.406: v199.14,77.83 203.4,77.83 206.25,74.98 206.25,66.65 204.01,64.41 204.01,64.01 JP6.11 | v190.19,77.22 190.19,76.61 v184.51,70.92 | v196.09,151.59 196.09,120.9 v206.25,110.74
REL32  (via drill 0.3)
  Top 0.406: 191.72,63.7 186.94,58.93 169.06,58.93 157.48,47.35 K25.1 | 191.72,63.7 191.82,63.8 201.37,63.8 JP6.12 | v149.96,137.57 145.9,137.57 142.24,133.91 142.24,105.66 v153.62,94.28 | v179.43,83.52 179.43,80.67 191.62,68.48 191.62,63.8 191.72,63.7
  Bottom 0.406: v149.96,137.57 157.68,145.29 160.32,145.29 K17.1 | v153.62,94.28 168.66,94.28 v179.43,83.52
REL33  (via drill 0.3)
  Top 0.406: v201.57,76.81 193.85,84.53 v182.88,84.53 | v146.91,93.27 124.77,93.27 124.56,93.07 80.47,93.07 71.53,102.01 71.53,104.04 52.83,122.73 48.56,122.73 40.84,115.01 40.84,114.81 29.26,103.23 28.25,103.23 K9.A2
  Bottom 0.406: v201.57,76.81 203.2,76.81 205.44,74.57 205.44,68.28 204.01,66.85 204.01,66.45 JP6.13 | v182.88,84.53 181.86,84.53 179.83,82.5 177.19,82.5 166.42,93.27 v146.91,93.27
REL34  (via drill 0.3)
  Top 0.406: v180.44,81.08 195.07,66.45 201.37,66.45 JP6.14 | v169.67,98.75 v169.67,88.59 | v159.51,98.75 153.62,92.86 148.34,92.86 141.02,85.55 141.02,74.57 135.74,69.29 87.78,69.29 84.53,66.04 77.01,66.04 56.9,86.16 v56.9,89.41
  Bottom 0.406: v180.44,81.08 177.19,81.08 v169.67,88.59 | v159.51,98.75 v169.67,98.75 | v56.9,89.41 41.86,104.44 41.86,104.85 35.97,110.74 28.25,110.74 K9.A1
REL35
  Top 0.406: JP6.15 204.01,69.09 204.01,69.49 205.44,70.92 205.44,74.57 188.16,91.85 182.88,91.85 173.53,101.19 K26.A2
REL36
  Top 0.406: JP6.16 201.37,69.09 196.9,69.09 173.53,92.46 173.53,93.67 K26.A1

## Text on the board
Bottom: SYNTUN1 | Helitron | V1.0
tNames: SYM TUNER / LC Board / DJ0ABR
